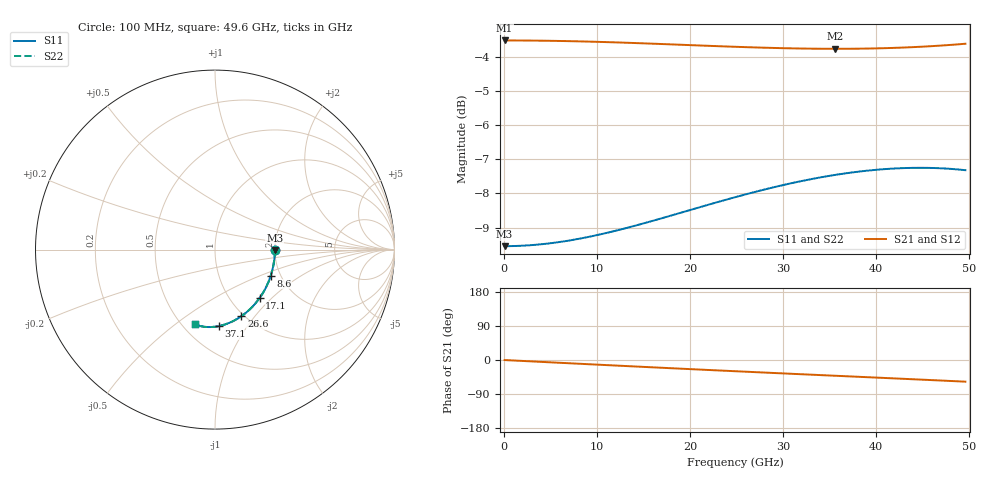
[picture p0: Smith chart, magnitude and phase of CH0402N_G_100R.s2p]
# GHz S RI R 100
! S-Parameters data
! Freq  reS11  imS11  reS21  imS21  reS12  imS12  reS22  imS22
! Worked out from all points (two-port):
!   100 points, 100 MHz to 49.6 GHz, reference 100 ohm
!   highest |S21| = -3.52 dB at 100 MHz (marker M1); lowest = -3.8 dB at 35.6 GHz (marker M2)
!   |S21| within 3 dB of the highest: start of sweep to end of sweep
!   lowest |S11| = -9.5 dB at 100 MHz (marker M3), VSWR 2.00, Z = 200 - j0.773 ohm
!   |S11| at or under -10 dB: nowhere
!   |S22| runs from -9.5 to -7.2 dB; largest |S21 - S12| = 0
!   S11 on the Smith chart (normalised r, x): 100 MHz: 2.00, -0.01; 8.6 GHz: 1.78, -0.58; 17.1 GHz: 1.36, -0.85; 26.6 GHz: 0.97, -0.86; 37.1 GHz: 0.72, -0.75; 49.6 GHz: 0.58, -0.59
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0.1  0.3333 -0.00172  0.6667 -0.00142  0.6667 -0.00142  0.3333 -0.00172
2.1  0.332 -0.036  0.6659 -0.0299  0.6659 -0.0299  0.332 -0.036
4.1  0.3282 -0.0701  0.6636 -0.0582  0.6636 -0.0582  0.3282 -0.0701
6.1  0.3219 -0.1036  0.6599 -0.0863  0.6599 -0.0863  0.3219 -0.1036
8.6  0.3109 -0.1444  0.6533 -0.1209  0.6533 -0.1209  0.3109 -0.1444
10.6  0.2995 -0.176  0.6465 -0.148  0.6465 -0.148  0.2995 -0.176
12.6  0.2861 -0.2063  0.6385 -0.1746  0.6385 -0.1746  0.2861 -0.2063
16.6  0.2536 -0.2625  0.6191 -0.2258  0.6191 -0.2258  0.2536 -0.2625
17.1  0.249 -0.269  0.6164 -0.232  0.6164 -0.232  0.249 -0.269
21.1  0.2094 -0.3173  0.5927 -0.2799  0.5927 -0.2799  0.2094 -0.3173
23.1  0.1877 -0.3385  0.5796 -0.3027  0.5796 -0.3027  0.1877 -0.3385
25.1  0.1651 -0.3577  0.5658 -0.3248  0.5658 -0.3248  0.1651 -0.3577
26.6  0.1476 -0.3706  0.5551 -0.3409  0.5551 -0.3409  0.1476 -0.3706
30.1  0.1056 -0.3959  0.529 -0.3769  0.529 -0.3769  0.1056 -0.3959
33.1  0.069 -0.4123  0.5054 -0.4063  0.5054 -0.4063  0.069 -0.4123
35.6  0.0385 -0.422  0.4851 -0.43  0.4851 -0.43  0.0385 -0.422
37.1  0.0204 -0.4262  0.4725 -0.4438  0.4725 -0.4438  0.0204 -0.4262
39.1  -0.00327 -0.4299  0.4555 -0.462  0.4555 -0.462  -0.00327 -0.4299
41.6  -0.032 -0.4316  0.4335 -0.4843  0.4335 -0.4843  -0.032 -0.4316
43.6  -0.054 -0.4305  0.4154 -0.5019  0.4154 -0.5019  -0.054 -0.4305
45.6  -0.0749 -0.4274  0.3967 -0.5194  0.3967 -0.5194  -0.0749 -0.4274
49.6  -0.1128 -0.4155  0.3573 -0.5541  0.3573 -0.5541  -0.1128 -0.4155
